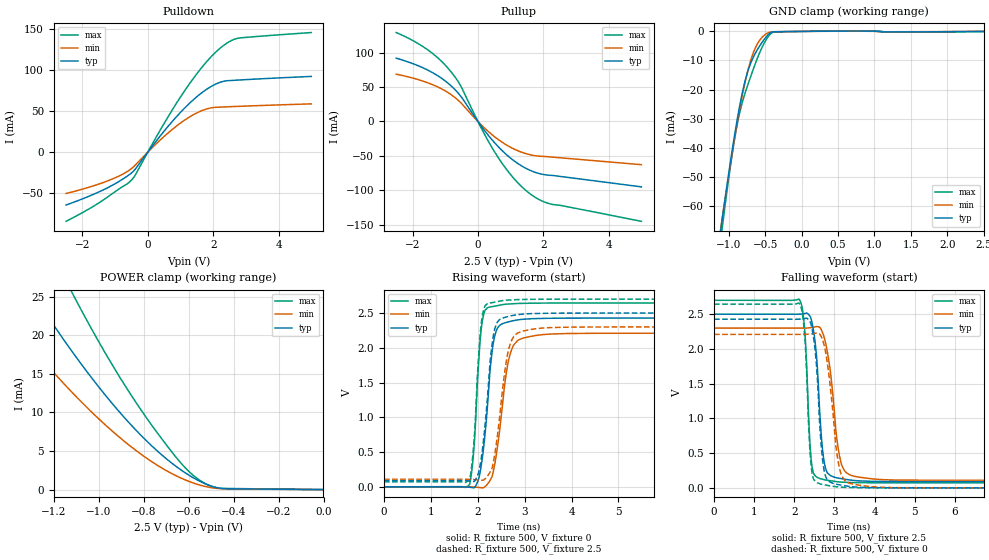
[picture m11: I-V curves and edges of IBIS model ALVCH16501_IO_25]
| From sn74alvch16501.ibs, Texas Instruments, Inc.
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[Model]   ALVCH16501_IO_25
Model_type  I/O
Vinl=0.7
Vinh=1.7
Enable   Active-Low
Vref =   0
Rref =   500
Cref =   30p
Vmeas =   1.25
| variable   typ   min   max
C_comp   3.08pF   2.52pF   3.40pF
| C_pullup   4.26pF   3.17pF   5.11pF
| C_pulldown   3.53pF   2.44pF   4.72pF
| C_tri-state   3.08pF   2.52pF   3.40pF
[Temperature Range]   40   100   -40
| Ambient temperature   25   85   -40
[Voltage range]   2.5   2.3   2.7
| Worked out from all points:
|   slope of the pulldown table from 0 to 0.375 V, typ, clamps not added: 19.2 ohm
|   slope of the pullup table from 0 to 0.375 V, typ, clamps not added: 16 ohm
|   GND clamp passes 1 mA (typ) near -0.45 V on its own axis
|   POWER clamp passes 1 mA (typ) near -0.54 V on its own axis
|   rising waveform, R_fixture 500, V_fixture 0: 20-80 % time 195ps typ, 251ps min, 136ps max; typ from 0 V to 2.43 V
|   falling waveform, R_fixture 500, V_fixture 2.5: 20-80 % time 166ps typ, 249ps min, 123ps max; typ from 2.5 V to 0.09 V
|   rising waveform, R_fixture 500, V_fixture 2.5: 20-80 % time 194ps typ, 243ps min, 135ps max; typ from 0.09 V to 2.5 V
|   falling waveform, R_fixture 500, V_fixture 0: 20-80 % time 164ps typ, 245ps min, 122ps max; typ from 2.43 V to 0 V
[GND Clamp]
| ALVCH16501_IO_25
|   Voltage   I(typ)   I(min)   I(max)
-2.5V     -353.4mA   -334.6mA   -384.6mA
-1.095V   -65.87mA   -65.51mA   -69mA
-1.08V    -63.15mA   -62.95mA   -66.02mA
-985mV    -46.48mA   -47.22mA   -48.05mA
-905mV    -33.64mA   -34.84mA   -35.07mA
-790mV    -18.62mA   -19.32mA   -22.5mA
-720mV    -12.44mA   -11.93mA   -17.14mA
-650mV    -8.288mA   -6.612mA   -12.16mA
-570mV    -4.833mA   -2.908mA   -7.059mA
-475mV    -1.597mA   -673.4uA   -2.431mA
-370mV    -112.8uA   -109.3uA   -161.9uA
2.5V      932.8pA    34.66uA    -62.19uA
[POWER Clamp]
| ALVCH16501_IO_25
|   Voltage   I(typ)   I(min)   I(max)
-2.5V     90.67mA    68.57mA    124.2mA
-1.49V    34.63mA    25.31mA    48.39mA
-1.465V   33.41mA    24.37mA    46.73mA
-1.295V   25.45mA    18.31mA    35.88mA
-1.275V   24.56mA    17.63mA    34.65mA
-1.115V   17.75mA    12.49mA    25.32mA
-965mV    12.04mA    8.233mA    17.4mA
-810mV    6.972mA    4.547mA    10.24mA
-655mV    2.988mA    1.783mA    4.157mA
-565mV    1.3mA      716.6uA    1.506mA
-455mV    155.4uA    121.3uA    164.2uA
-31.15fV  932.8pA    48.41nA    38.21pA
[Pulldown]
| ALVCH16501_IO_25
|   Voltage   I(typ)   I(min)   I(max)
-2.5V     -64.59mA   -50.56mA   -84.54mA
-1.23V    -43.52mA   -35.16mA   -54.83mA
-790mV    -33.54mA   -27.38mA   -42.65mA
-485mV    -25mA      -19.64mA   -33.5mA
-380mV    -20.56mA   -15.66mA   -27.74mA
450mV     23.28mA    17.43mA    31.8mA
1.14V     54.41mA    39.51mA    75.81mA
1.745V    75.37mA    52.1mA     108mA
2.295V    86.37mA    55.21mA    129.8mA
2.555V    87.66mA    55.65mA    136.4mA
2.795V    88.23mA    56.04mA    139.6mA
5V        92.59mA    59.04mA    146.2mA
[Pullup]
| ALVCH16501_IO_25
|   Voltage   I(typ)   I(min)   I(max)
-2.5V     91.82mA    68.58mA    129mA
-1.555V   74.97mA    56.45mA    104.6mA
-1.18V    64.82mA    48.92mA    90.2mA
-855mV    53.1mA     40.01mA    73.9mA
-535mV    37.16mA    27.63mA    52.24mA
140mV     -9.241mA   -6.718mA   -13.1mA
595mV     -35.26mA   -25.25mA   -50.51mA
1.08V     -56.23mA   -39.45mA   -81.67mA
1.565V    -70.25mA   -47.93mA   -103.9mA
1.89V     -75.76mA   -50.41mA   -113.8mA
2.215V    -78.17mA   -51.5mA    -119.6mA
5V        -94.9mA    -62.72mA   -144.9mA
[Ramp]
| ALVCH16501_IO_25
| variable   typ   min   max
dV/dt_r   1.47/2.07E-10   1.33/2.75E-10   1.59/1.41E-10
dV/dt_f   1.46/1.74E-10   1.33/2.67E-10   1.59/1.26E-10
R_load = 500
[Rising Waveform]
| ALVCH16501_IO_25
R_fixture =   500
C_fixture =   0
L_fixture =   0
V_fixture =   0
V_fixture_min = 0
V_fixture_max = 0
|   Time   V(typ)   V(min)   V(max)
0s        86.95pV    2.936nV    67.35pV
1.825ns   -6.64mV    260.2uV    33.22mV
1.92ns    -14.79mV   -3.293mV   560.8mV
2.035ns   156.7mV    -10.79mV   1.953V
2.11ns    479mV      -15.45mV   2.429V
2.34ns    2.099V     248.2mV    2.596V
2.63ns    2.369V     1.723V     2.628V
2.875ns   2.403V     2.114V     2.638V
3.895ns   2.426V     2.205V     2.644V
50ns      2.428V     2.209V     2.645V
[Falling Waveform]
| ALVCH16501_IO_25
R_fixture =   500
C_fixture =   0
L_fixture =   0
V_fixture =   2.5
V_fixture_min = 2.3
V_fixture_max = 2.7
|   Time   V(typ)   V(min)   V(max)
0s        2.5V       2.3V       2.7V
2.125ns   2.5V       2.299V     2.711V
2.27ns    2.511V     2.299V     2.186V
2.385ns   2.475V     2.305V     678.7mV
2.455ns   2.338V     2.31V      259.9mV
2.555ns   1.888V     2.323V     158mV
2.745ns   367.7mV    2.163V     117.9mV
3.125ns   137mV      461mV      85.08mV
4.605ns   90.49mV    111.4mV    72.15mV
50ns      89.71mV    108.1mV    72.01mV
[Rising Waveform]
| ALVCH16501_IO_25
R_fixture =   500
C_fixture =   0
L_fixture =   0
V_fixture =   2.5
V_fixture_min = 2.3
V_fixture_max = 2.7
|   Time   V(typ)   V(min)   V(max)
0s        89.71mV    108.1mV    72.01mV
1.825ns   82.97mV    107.4mV    106.9mV
1.92ns    76.14mV    103.9mV    647.4mV
2.025ns   221.8mV    97.85mV    1.951V
2.105ns   567.4mV    94.2mV     2.487V
2.335ns   2.184V     361.9mV    2.653V
2.615ns   2.444V     1.828V     2.685V
2.855ns   2.477V     2.214V     2.693V
3.87ns    2.499V     2.296V     2.7V
50ns      2.5V       2.3V       2.7V
[Falling Waveform]
| ALVCH16501_IO_25
R_fixture =   500
C_fixture =   0
L_fixture =   0
V_fixture =   0
V_fixture_min = 0
V_fixture_max = 0
|   Time   V(typ)   V(min)   V(max)
0s        2.428V     2.209V     2.645V
2.125ns   2.428V     2.209V     2.654V
2.265ns   2.438V     2.209V     2.135V
2.385ns   2.397V     2.214V     570.2mV
2.45ns    2.264V     2.219V     185.5mV
2.73ns    292mV      2.08V      45.64mV
3.095ns   47mV       368.9mV    12.85mV
3.365ns   21.56mV    69.61mV    5.011mV
4.49ns    828.9uV    3.138mV    171.6uV
50ns      363.7pV    4.023nV    -931.2pV
